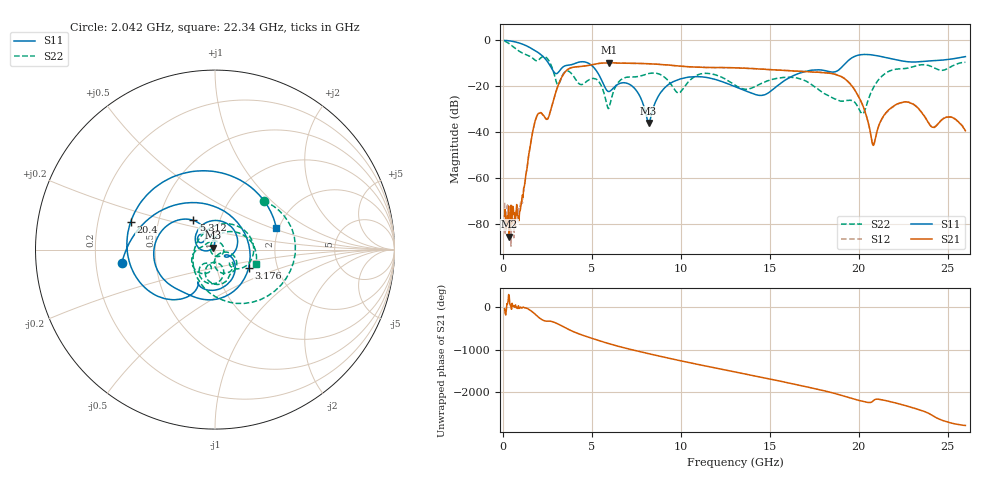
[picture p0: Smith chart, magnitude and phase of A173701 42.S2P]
!  2-Port S-parameters saved by WinCal
! VAR MeasName=S-Parameters (CALIBRATED_DATA) read from VNA (N5245A)
! VAR MeasDate=2017-6-7 10:31:13
! VAR NAME=A173701 42
! VAR FILENAME=A173701 42.S2P
! VAR DATE=2017-6-7 10:31:13
! VAR PHYS_PORTS=1,2
# Hz S DB R 50
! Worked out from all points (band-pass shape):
!   801 points, 100 MHz to 26 GHz, reference 50 ohm
!   highest |S21| = -9.75 dB at 5.96 GHz (marker M1); lowest = -85.5 dB at 359 MHz (marker M2)
!   |S21| within 3 dB of the highest: 3.635 GHz to 15.03 GHz (11.39 GHz wide, 122 % of centre)
!   lowest |S11| = -36.0 dB at 8.194 GHz (marker M3), VSWR 1.03, Z = 48.8 + j1.02 ohm
!   |S11| at or under -10 dB: 2.575 GHz to 4.07 GHz (1.495 GHz wide, 45 % of centre); 4.827 GHz to 19.25 GHz (14.43 GHz wide, 120 % of centre)
!   |S22| runs from -32.0 to -0.2 dB; largest |S21 - S12| = 0.0045
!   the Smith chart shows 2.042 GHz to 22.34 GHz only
!   S11 on the Smith chart (normalised r, x): 2.042 GHz: 0.31, -0.06; 3.176 GHz: 1.42, -0.31; 5.312 GHz: 0.75, +0.25; 20.4 GHz: 0.35, +0.14; 22.34 GHz: 1.94, +0.53
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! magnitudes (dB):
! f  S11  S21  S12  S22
! 100 MHz  0.0  -76.6  -70.8  -0.2
! 359 MHz  -0.2  -85.5  -80.1  -1.4
! 974.1 MHz  -1.3  -74.3  -72.4  -5.0
! 2.042 GHz  -5.6  -31.8  -31.8  -8.3
! 2.528 GHz  -9.5  -34.2  -34.2  -8.2
! 3.176 GHz  -13.4  -18.3  -18.3  -18.7
! 4.438 GHz  -9.3  -11.3  -11.3  -19.3
! 5.312 GHz  -13.9  -10.1  -10.2  -17.3
! 5.96 GHz  -22.3  -9.8  -9.8  -29.5
! 7.223 GHz  -19.6  -10.0  -10.0  -16.0
! 8.194 GHz  -36.0  -10.1  -10.1  -14.5
! 8.744 GHz  -24.3  -10.4  -10.4  -14.5
! 9.845 GHz  -17.1  -11.1  -11.1  -22.9
! 11.24 GHz  -15.9  -11.7  -11.8  -14.4
! 13.05 GHz  -20.1  -12.0  -12.0  -19.5
! 17.39 GHz  -12.9  -13.8  -13.6  -19.4
! 19.27 GHz  -9.9  -17.0  -16.9  -26.3
! 20.4 GHz  -6.1  -32.0  -32.1  -29.4
! 20.82 GHz  -6.4  -45.8  -46.0  -20.8
! 21.69 GHz  -7.8  -30.2  -30.4  -13.5
! 22.34 GHz  -8.8  -27.2  -27.3  -12.4
! 26 GHz  -7.1  -39.4  -39.4  -9.5
